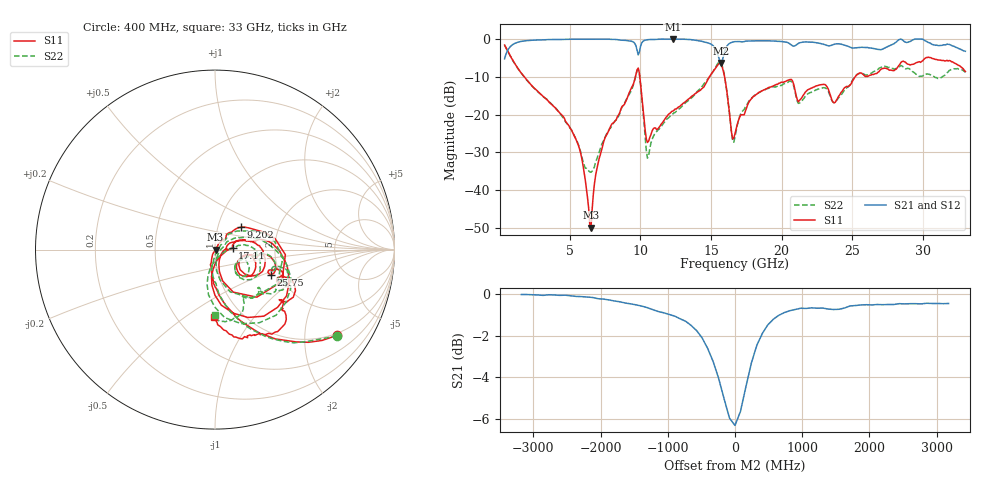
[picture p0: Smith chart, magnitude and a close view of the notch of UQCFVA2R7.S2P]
!  Part Number  UQCFVA2R7  Mounting Orientation: Horizontal
!  Description: Ultra Low ESR Microwave capacitors
!  Application: Coupling, Bypass, Tuning, DC Block
!  Filters, Matching
# GHZ S DB R 50
! Freq  |S11|  S11 Ph  |S21|  S21 Ph  |S12|  S12 Ph  |S22|  S22 Ph
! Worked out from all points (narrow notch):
!   401 points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, 400 MHz to 33 GHz, reference 50 ohm
!   highest |S21| = 0.00 dB at 12.3 GHz (marker M1); lowest = -6.3 dB at 15.72 GHz (marker M2)
!   notch at M2: 5.7 dB deep, 533 MHz wide at half that depth
!   lowest |S11| = -50.0 dB at 6.513 GHz (marker M3), VSWR 1.01, Z = 50.3 + j0.0349 ohm
!   |S11| at or under -10 dB: 1.794 GHz to 9.651 GHz (7.857 GHz wide, 137 % of centre); 9.964 GHz to 14.89 GHz (4.926 GHz wide, 39.6 % of centre); 15.96 GHz to 25.2 GHz (9.24 GHz wide, 44.9 % of centre)
!   |S22| runs from -35.3 to -1.6 dB; largest |S21 - S12| = 0.014
!   S11 on the Smith chart (normalised r, x): 400 MHz: 0.93, -2.90; 9.202 GHz: 1.29, +0.33; 17.11 GHz: 1.22, +0.02; 25.75 GHz: 1.79, -0.56; 33 GHz: 0.75, -0.65
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0.4  -1.59 -35.0  -5.22 54.8  -5.22 54.7  -1.58 -35.2
1.786  -9.96 -79.0  -0.50 10.4  -0.49 10.3  -10.06 -79.4
4.475  -20.21 -103.2  -0.08 -13.5  -0.09 -13.6  -20.54 -100.1
5.861  -31.65 -116.8  -0.02 -22.5  -0.02 -22.5  -31.14 -87.0
6.513  -49.98 6.3  -0.03 -26.4  -0.03 -26.5  -35.30 -17.5
7.409  -27.20 56.4  -0.04 -32.2  -0.04 -32.2  -26.87 40.5
9.202  -14.36 40.8  -0.46 -45.2  -0.45 -45.1  -14.71 34.7
9.854  -7.68 -25.4  -4.19 -44.7  -4.10 -44.5  -8.07 -29.2
10.506  -27.41 -33.1  -0.17 -41.1  -0.19 -41.1  -31.57 -32.7
11.321  -23.42 14.9  -0.03 -48.4  -0.02 -48.4  -23.88 28.3
12.299  -19.07 22.3  0.00 -56.2  0.00 -56.2  -19.84 31.9
14.826  -10.42 8.7  -1.05 -77.9  -1.04 -77.9  -10.43 5.1
15.722  -6.74 -53.7  -6.32 -66.6  -6.21 -66.9  -6.44 -58.9
16.7  -25.11 -16.4  -0.67 -66.1  -0.70 -66.0  -25.91 -18.1
17.108  -20.09 4.3  -0.71 -70.8  -0.69 -70.7  -19.76 4.1
19.797  -11.71 1.5  -0.59 -90.3  -0.61 -90.3  -12.44 -8.0
22.161  -12.93 -15.4  -0.81 -101.5  -0.81 -101.6  -13.98 -23.7
23.791  -16.78 -21.9  -1.31 -108.2  -1.30 -108.1  -16.66 -27.7
25.747  -9.34 -24.0  -2.19 -117.9  -2.18 -117.5  -9.14 -19.3
27.621  -8.26 -27.1  -1.81 -118.2  -1.78 -118.0  -7.51 -25.2
29.985  -5.72 -41.5  -0.04 -151.4  -0.07 -151.2  -9.75 -40.6
33  -8.57 -90.6  -3.23 -170.0  -3.19 -169.7  -8.81 -89.7
